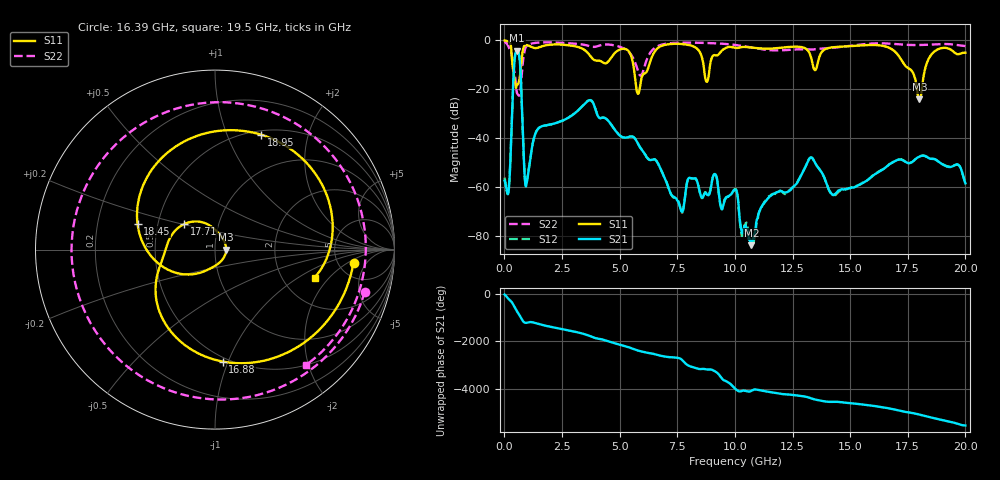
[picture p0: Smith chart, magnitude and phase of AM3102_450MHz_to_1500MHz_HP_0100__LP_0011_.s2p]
!Agilent Technologies,E8364B,MY43040894,A.07.50.67
!Agilent E8364B: A.07.50.67
!Date: Thursday, January 11, 2018 05:35:57
!Correction: S11(Full 2 Port(1,2))
!S21(Full 2 Port(1,2))
!S12(Full 2 Port(1,2))
!S22(Full 2 Port(1,2))
!S2P File: Measurements: S11, S21, S12, S22:
# Hz S  dB  R 50
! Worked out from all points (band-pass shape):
!   1601 points, 10 MHz to 20 GHz, reference 50 ohm
!   highest |S21| = -4.26 dB at 547.2 MHz (marker M1); lowest = -83.8 dB at 10.72 GHz (marker M2)
!   |S21| within 3 dB of the highest: 450.4 MHz to 658.2 MHz (207.7 MHz wide, 37.5 % of centre)
!   lowest |S11| = -24.1 dB at 18 GHz (marker M3), VSWR 1.13, Z = 56.6 - j0.0242 ohm
!   |S11| at or under -10 dB: 352 MHz to 730 MHz (378.1 MHz wide, 69.9 % of centre); 5.591 GHz to 6.284 GHz (693.1 MHz wide, 11.7 % of centre); 17.35 GHz to 18.3 GHz (949.4 MHz wide, 5.33 % of centre)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
!   |S22| runs from -22.6 to -0.6 dB; largest |S21 - S12| = 0.003
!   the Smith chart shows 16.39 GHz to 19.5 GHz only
!   S11 on the Smith chart (normalised r, x): 16.39 GHz: 6.96, -2.54; 16.88 GHz: 0.47, -0.95; 17.71 GHz: 0.68, +0.21; 18.45 GHz: 0.38, +0.14; 18.95 GHz: 0.55, +1.33; 19.5 GHz: 3.00, -1.40
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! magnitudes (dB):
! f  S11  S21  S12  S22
! 10 MHz  -0.1  -57.4  -56.1  -0.6
! 184.9 MHz  -0.6  -61.6  -60.8  -2.8
! 547.2 MHz  -18.3  -4.3  -4.3  -21.6
! 959.5 MHz  -2.0  -58.9  -58.8  -2.4
! 1.459 GHz  -3.0  -36.2  -36.2  -0.9
! 3.346 GHz  -3.3  -27.3  -27.3  -1.7
! 5.807 GHz  -21.9  -42.5  -42.5  -12.9
! 6.682 GHz  -3.0  -50.7  -50.7  -2.3
! 7.694 GHz  -1.5  -70.1  -70.5  -1.0
! 10.01 GHz  -3.1  -61.0  -60.9  -1.9
! 10.72 GHz  -2.9  -83.8  -84.1  -2.9
! 13.34 GHz  -8.4  -48.1  -48.0  -3.8
! 14.28 GHz  -2.8  -63.3  -63.4  -3.1
! 16.39 GHz  -2.2  -53.0  -52.9  -1.2
! 16.68 GHz  -3.0  -50.9  -50.9  -1.3
! 16.88 GHz  -4.1  -49.8  -49.7  -1.5
! 17.71 GHz  -13.1  -49.6  -49.6  -1.9
! 18 GHz  -24.1  -47.6  -47.6  -1.9
! 18.45 GHz  -6.8  -48.4  -48.3  -1.7
! 18.95 GHz  -3.2  -50.4  -50.3  -1.5
! 19.5 GHz  -4.8  -51.3  -51.2  -1.7
! 20 GHz  -5.1  -58.5  -58.3  -2.4
